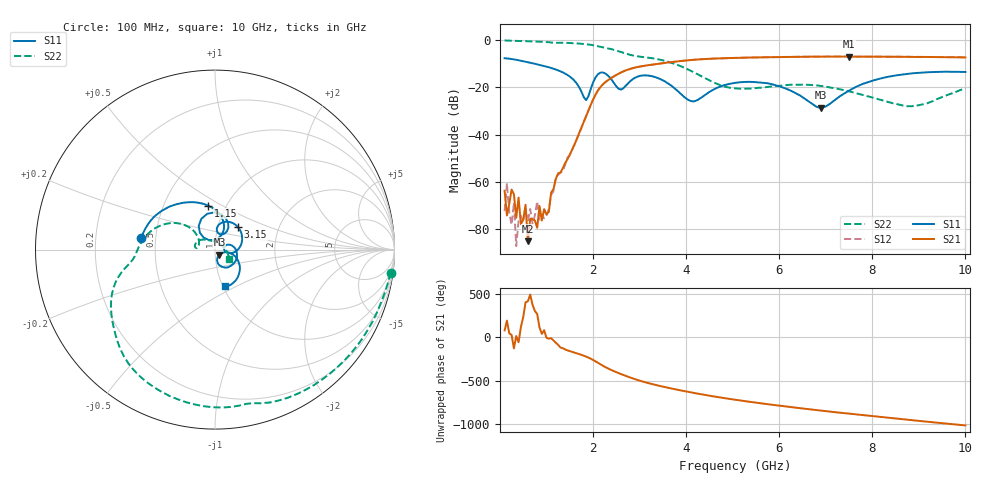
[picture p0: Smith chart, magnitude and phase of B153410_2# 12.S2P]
!  2-Port S-parameters saved by WinCal
! VAR MeasName=S-Parameters (CALIBRATED_DATA) read from VNA (N5245A)
! VAR MeasDate=2016-12-23 9:59:57
! VAR NAME=B153410_2# 12
! VAR FILENAME=B153410_2# 12.S2P
! VAR DATE=2016-12-23 9:59:57
! VAR PHYS_PORTS=1,2
# Hz S DB R 50
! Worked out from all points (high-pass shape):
!   199 points, 100 MHz to 10 GHz, reference 50 ohm
!   highest |S21| = -6.95 dB at 7.5 GHz (marker M1); lowest = -85.3 dB at 600 MHz (marker M2)
!   |S21| within 3 dB of the highest: 3.428 GHz to end of sweep
!   lowest |S11| = -28.6 dB at 6.9 GHz (marker M3), VSWR 1.08, Z = 52.4 - j2.9 ohm
!   |S11| at or under -10 dB: 748.5 MHz to end of sweep
!   |S22| runs from -28.0 to -0.1 dB; largest |S21 - S12| = 0.0033
!   S11 on the Smith chart (normalised r, x): 100 MHz: 0.42, +0.06; 1.15 GHz: 0.82, +0.43; 3.15 GHz: 1.25, +0.32; 10 GHz: 1.02, -0.44
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1e8  -7.64 171.4  -63.80 78.3  -72.42 110.7  -0.12 -7.5
1.5e8  -7.72 167.1  -74.29 -169.1  -60.56 174.3  -0.16 -10.9
2.5e8  -7.99 158.8  -63.29 26.9  -78.21 138.5  -0.25 -17.6
3e8  -8.15 155.0  -65.32 -129.1  -68.83 -2.8  -0.28 -21.0
3.5e8  -8.31 151.1  -75.23 12.5  -87.29 24.0  -0.31 -24.3
4e8  -8.51 147.5  -66.71 -59.2  -76.64 -179.2  -0.34 -27.6
4.5e8  -8.70 144.0  -77.96 117.6  -74.46 150.6  -0.36 -30.9
5.5e8  -9.11 137.1  -69.74 42.3  -72.09 -163.2  -0.42 -37.5
6e8  -9.35 133.9  -85.28 54.1  -76.68 149.9  -0.45 -40.8
1e9  -11.21 108.8  -73.85 -7.8  -74.54 43.9  -0.79 -67.0
1.15e9  -12.10 99.1  -63.14 -38.0  -63.97 -32.5  -1.10 -76.1
1.75e9  -21.80 67.6  -37.06 156.7  -37.17 157.1  -1.52 -113.5
2.2e9  -13.66 90.9  -18.96 33.6  -18.95 33.8  -2.96 -142.6
3.15e9  -14.93 44.3  -10.71 -164.2  -10.73 -164.1  -7.33 179.7
3.4e9  -16.11 16.5  -10.02 161.9  -10.03 162.2  -8.11 169.1
4.15e9  -25.97 5.7  -8.33 78.4  -8.33 78.6  -13.47 140.6
5.05e9  -18.10 -10.7  -7.50 -1.5  -7.51 -1.3  -20.42 159.4
6.7e9  -26.96 -71.4  -6.98 -114.8  -6.98 -114.7  -19.00 160.0
6.9e9  -28.63 -48.2  -6.97 -127.1  -6.97 -127.0  -19.43 154.4
7.5e9  -21.40 -12.6  -6.95 -162.5  -6.96 -162.4  -21.72 137.3
8.35e9  -15.47 -34.7  -7.03 149.7  -7.01 150.0  -26.27 104.6
1e10  -13.48 -75.3  -7.31 61.9  -7.28 62.3  -20.44 -33.4
